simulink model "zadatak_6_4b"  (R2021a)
settings: Solver=VariableStepAuto  StartTime=0.0  StopTime=0.5  RelTol=1e-3
libraries: spsGroundLib x2, spsVoltageMeasurementLib x2, spsDistributedParametersLineLib x1, spsThreePhaseSourceLib x1, spsThreePhaseBreakerLib x1, spsThreePhaseSeriesRLCLoadLib x1, spspowerguiLib x1

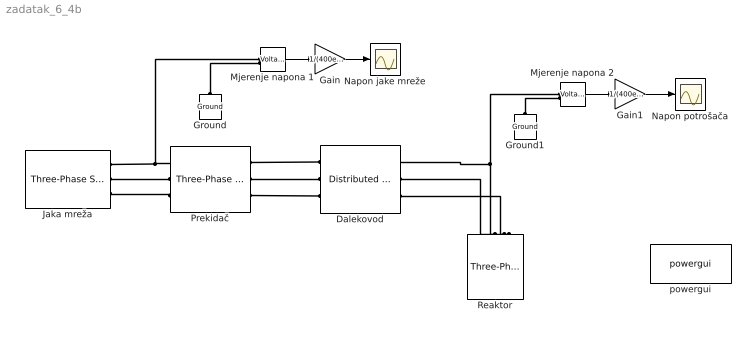
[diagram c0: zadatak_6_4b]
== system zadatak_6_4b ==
  Dalekovod : spsDistributedParametersLineLib/Distributed Parameters Line  Phases=3  Length=100  Frequency=50  Resistance=[0.011 0.3864]  Inductance="[0.8675e-3  4.1264e-3]"  Capacitance=[13.41e-9 7.751e-9]  x1=[3.77109743319994e-10 2.9241229649179e-10 5.74831442464142e-11;314.159265358979 314.159265358979 314.159265358979;1.36136989538347 1.45402689054562 1.45402689054564]  x2=[3.5136976526336e-10 2.88668769659188e-10 5.67472323320025e-11;314.159265358979 314.159265358979 314.159265358979;1.381194858386 1.45448040499324 1.45448040499327]  x3=[5.13988740012816e-13 1.14772788256905e-12 2.2562323206268e-13;314.159265358979 314.159265358979 314.159265358979;1.65465859779076 1.52009849441941 1.52009849441945]  x4=[5.19909496560205e-13 1.14913444994705e-12 2.25899738613369e-13;314.159265358979 314.159265358979 314.159265358979;0.911639251404753 1.28128517482317 1.28128517482319]  x5=0.000565541566995742  V1=[3.771e-10 2.924e-10 5.748e-11;314.2 314.2 314.2;1.361 1.454 1.454]  V2=[3.514e-10 2.887e-10 5.675e-11;314.2 314.2 314.2;1.381 1.454 1.454]  I1=[5.14e-13 1.148e-12 2.256e-13;314.2 314.2 314.2;1.655 1.52 1.52]  I2=[5.199e-13 1.149e-12 2.259e-13;314.2 314.2 314.2;0.9116 1.281 1.281]  nHarmo=1  Measurements=None  Decoupling=off  VsMag0=0  VrMag0=0  VsAngle0=0  VrAngle0=0  IsMag0=0  IrMag0=0  IsAngle0=0  IrAngle0=0
  Gain : Gain  Gain=1/(400e3/sqrt(3)*sqrt(2))
  Gain1 : Gain  Gain=1/(400e3/sqrt(3)*sqrt(2))
  Ground : spsGroundLib/Ground  LConnTagsString=a
  Ground1 : spsGroundLib/Ground  LConnTagsString=a
  Jaka mreža : spsThreePhaseSourceLib/Three-Phase Source  InternalConnection=Yg  VoltagePhases=off  Voltage=(400000)*1.00018  PhaseAngle=0.00047733  Voltage_phases=[25e3 25e3 25e3]/sqrt(3)  PhaseAngles_phases=[0 -120 +120]  Frequency=50  NonIdealSource=on  SpecifyImpedance=off  Resistance=180.1  Inductance=26.525e-3  ShortCircuitLevel=100e6  BaseVoltage=400e3  XRratio=7  BusType=swing  Pref=10000  Qref=0  Prefabc=[10e3, 10e3, 10e3]  Qrefabc=[0, 0, 0]  Qmin=-Inf  Qmax=Inf
  Mjerenje napona 1 : spsVoltageMeasurementLib/Voltage Measurement  PhasorSimulation=off  OutputType=Complex  PSBequivalent=0
  Mjerenje napona 2 : spsVoltageMeasurementLib/Voltage Measurement  PhasorSimulation=off  OutputType=Complex  PSBequivalent=0
  Napon jake mreže : Scope
  Napon potrošača : Scope
  Prekidač : spsThreePhaseBreakerLib/Three-Phase Breaker  InitialState=open  SwitchA=on  SwitchB=on  SwitchC=on  SwitchTimes=[25e-3]  External=off  BreakerResistance=0.01  SnubberResistance=inf  SnubberCapacitance=inf  Measurements=None
  Reaktor : spsThreePhaseSeriesRLCLoadLib/Three-Phase Series RLC Load  LConnTagsString=A|B|C  Configuration=Y (grounded)  NominalVoltage=400e3  Vabc=[1e3 1e3 1e3]  Vabcp=[1e3 1e3 1e3]  NominalFrequency=50  UnbalancedPower=off  ActivePower=366666.6667  InductivePower=110000000  CapacitivePower=0  Pabc=[10e3 9e3 11e3]  QLabc=[100 90 110]  QCabc=[100 90 110]  Pabcp=[10e3 9e3 11e3]  QLabcp=[100 90 110]  QCabcp=[100 90 110]  Measurements=None  LoadType=constant Z
  powergui : spspowerguiLib/powergui  Priority=1  SimulationMode=Continuous  SampleTime=50e-6  frequency=60  Iterations=50  frequencyindice=50  Pbase=100e6  ErrMax=1e-4  UnitsV=kV  UnitsW=MW  buscounter=0  FunctionMessages=off  echomessages=off  EnableUseOfTLC=off  CurrentSourceSwitches=off  DisableSnubberDevices=off  DisableRonSwitches=off  DisableVfSwitches=off  DisplayEquations=off  AutomaticDiscreteSolvers=off  SolverType=Tustin/Backward Euler (TBE)  Interpol=off  ExternalGateDelay=off  methode=off  Ts=100  x0status=blocks  SPID=on  SwTol=0  HookPort=off  NonlinearTolerance=1e-4  nMaxIteration=100  ContinueOnMaxIteration=off  RestoreLinks=warning  ResistiveCurrentMeasurement=off  Frange=[0:2:500]  Ylog=off  Xlog=on  ShowGrid=off  save=off  variable=ZData  structure=0  ZoomFFT=off  StartTime=0.0  cycles=1  DisplayStyle=1  fundamental=60  FreqAxis=off  MaxFrequency=1000  frequencyindicesteady=1  RmsSteady=1  display=off
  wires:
  Gain/1 -> Napon jake mreže/1
  Mjerenje napona 1/1 -> Gain/1
  Mjerenje napona 2/1 -> Gain1/1
  Gain1/1 -> Napon potrošača/1
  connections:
  Mjerenje napona 1/LConn1 -- Jaka mreža/RConn1 -- Prekidač/LConn1
  Mjerenje napona 2/LConn1 -- Dalekovod/RConn1 -- Reaktor/LConn1
  Dalekovod/RConn2 -- Reaktor/LConn2
  Dalekovod/RConn3 -- Reaktor/LConn3
  Ground/LConn1 -- Mjerenje napona 1/LConn2
  Ground1/LConn1 -- Mjerenje napona 2/LConn2
  Dalekovod/LConn1 -- Prekidač/RConn1
  Dalekovod/LConn2 -- Prekidač/RConn2
  Dalekovod/LConn3 -- Prekidač/RConn3
  Prekidač/LConn2 -- Jaka mreža/RConn2
  Prekidač/LConn3 -- Jaka mreža/RConn3
